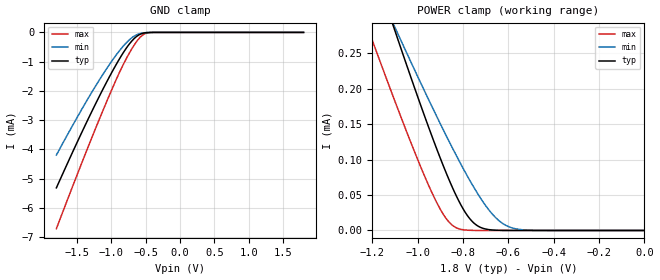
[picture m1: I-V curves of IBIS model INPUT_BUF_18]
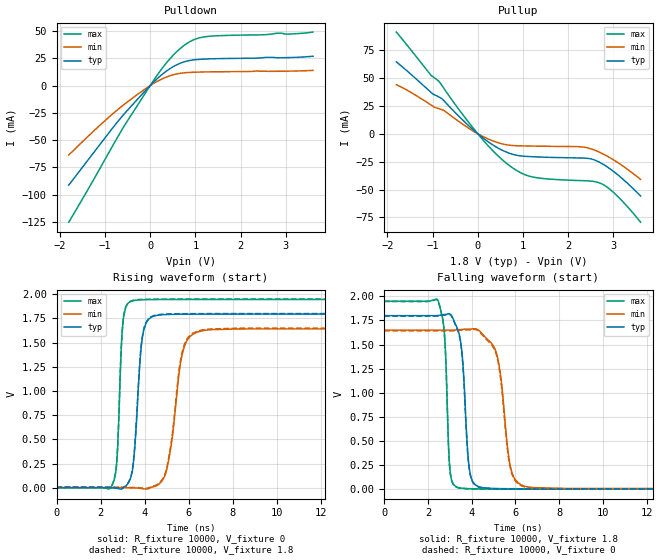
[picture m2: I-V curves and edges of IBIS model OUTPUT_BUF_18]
| TEXAS INSTRUMENTS INCORPORATED
| DLP Products
| IBIS Model of D3664YV2DL
| DLP2000 DMD
| This file contains package information for the following:
|  - LGA 42-pin (PW) package as [Component] DLP2000 DMD
| This device can be powered at the following Vccs:
|  1.8 volt Vcc
| This file provides unique models under the [Model Selector] for each Vcc.
| For operation at a specific Vcc, select the appropriate model after each
| [Model Selector] keyword.
[IBIS Ver]   3.2
[Comment char]  |_char
[File Name]   dlp2000dmd_ibis.ibs
[File Rev]   1.0 | f_die
[Date]   October 20, 2009
[Source]   Data created from TI-SPICE simulations at TI-SLL.
[Notes]   The following is an IBIS list for the P22_NHD.
   Please contact sllibis@ti.com with questions and
   comments concerning SLL IBIS models.
##notes##|
[Disclaimer] Property of Texas Instruments Incorporated.  Unauthorized
   reproduction and/or distribution is strictly prohibited.
   This product is protected under copyright law.
   Created  2009, (C) Copyright  2009, Texas Instruments
   Incorporated, All Rights Reserved
   UNLESS THERE IS A SIGNED, WRITTEN AGREEMENT TO THE
   CONTRARY, TEXAS INSTRUMENTS (TI) IS PROVIDING THE IBIS
   MODELS  AND WITHOUT ANY WARRANTY, EXPRESSED OR
   IMPLIED.  TI assumes no liability for:
   1) the accuracy of the IBIS models provided to your
   company;
   2) the proper functioning of these IBIS Models in your
   design or for any resulting applications; or
   3) infringement of patents, copyrights or intellectual
   property rights resulting from your use of these IBIS
   models.
   TI provides IBIS Models as a service to our customers.
   You and your company shall not distribute, sell or give
   these models to anyone else without prior written
   permission from TI.
   TI reserves the right to make changes to our products or
   to discontinue any semiconductor product or service
   without notice, and advises our customers to obtain the
   latest version of relevant information to verify, before
   placing orders, that the information being relied on is
   current.
   Please be aware that your receipt and use of the IBIS
   information provided shall serve as acceptance of these
   terms and conditions.  If you do not accept these terms,
   you should return or destroy the IBIS models and any
   other accompanying information immediately.
| Component DLP2000 42-pin - LGA
[Component]   DLP2000
[Manufacturer]   Texas Instruments, Inc.
[Package]
|   typ   min   max
R_pkg   6.280e-01   1.680e-01   1.260e+00
L_pkg   5.240e-09   2.810e-09   7.630e-09
C_pkg   2.160e-12   1.040e-12   4.000e-12
[Pin]   signal_name   model_name   R_pin   L_pin   C_pin
1   VCC   POWER
2   D<1>   INPUT_BUF
3   VSS   GND
4   D<2>   INPUT_BUF
5   VSS   GND
6   D<3>   INPUT_BUF
7   D<4>   INPUT_BUF
8   D<5>   INPUT_BUF
9   VSS   GND
10   D<7>   INPUT_BUF
11   VCC   POWER
12   D<6>   INPUT_BUF
13   D<0>   INPUT_BUF
14   VSS   GND
15   DAD_STROBE INPUT_BUF
16   VBIAS   POWER
17   VSS   GND
18   VSS   GND
19   VSS   GND
20   VRESET   POWER
21   VCC   POWER
22   VCC   POWER
23   D<9>   INPUT_BUF
24   VSS   GND
25   D<8>   INPUT_BUF
26   VSS   GND
27   D<11>   INPUT_BUF
28   D<10>   INPUT_BUF
29   VSS   GND
30   DCLK   INPUT_BUF
31   LOADB   INPUT_BUF
32   VCC   POWER
33   SCTRL   INPUT_BUF
34   VSS   GND
35   DAD_BUS   INPUT_BUF
36   VOFFSET   POWER
37   SAC_BUS   INPUT_BUF
38   VSS   GND
39   DAD_OEZ   INPUT_BUF
40   VSS   GND
41   SCAN_TEST  OUTPUT_BUF
42   VCC   POWER
| Model INPUT_BUF
[Model Selector]   INPUT_BUF
INPUT_BUF_18   1.8 volt Vcc
| Model OUTPUT_BUF
[Model Selector]   OUTPUT_BUF
OUTPUT_BUF_18   1.8 volt Vcc
| Models and submodels in the file (2): INPUT_BUF_18 (Input), OUTPUT_BUF_18 (Output)
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[Model]   INPUT_BUF_18
Model_type  Input
Vinl = 0.55
Vinh = 1.25
| variable   typ   min   max
C_comp   0.28pF   0.24pF   0.33pF
[Temperature Range]   40   100   -40
| Ambient temperature   25   85   -40
[Voltage range]   1.8   1.65   1.95
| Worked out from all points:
|   GND clamp passes 1 mA (typ) near -0.90 V on its own axis
[GND Clamp]
| INPUT_BUF_18
|   Voltage   I(typ)   I(min)   I(max)
-1.8V     -5.319mA   -4.198mA   -6.715mA
-1.555V   -4.052mA   -3.147mA   -5.216mA
-1.335V   -2.953mA   -2.248mA   -3.902mA
-1.14V    -2.026mA   -1.501mA   -2.773mA
-970mV    -1.27mA    -905.4uA   -1.833mA
-850mV    -785.1uA   -536.1uA   -1.214mA
-735mV    -390.1uA   -249.6uA   -697.8uA
-640mV    -155uA     -91.95uA   -339.3uA
-555mV    -40.52uA   -24.77uA   -113.2uA
-485mV    -8.678uA   -6.212uA   -26.14uA
-385mV    -582.9nA   -605.8nA   -1.321uA
1.8V      14.91pA    71.9pA     7.535pA
[POWER Clamp]
| INPUT_BUF_18
|   Voltage   I(typ)   I(min)   I(max)
-1.8V     972.9uA    792.1uA    806.9uA
-1.22V    396.3uA    370.8uA    285.3uA
-1.11V    290.7uA    293.1uA    190.3uA
-1.095V   276.5uA    282.7uA    177.6uA
-930mV    126.7uA    170.1uA    48.3uA
-875mV    81.58uA    134.2uA    17uA
-830mV    48.86uA    105.9uA    3.835uA
-785mV    22.91uA    79.02uA    514nA
-740mV    7.387uA    54.23uA    58.41nA
-670mV    665.1nA    22.78uA    1.924nA
-600mV    46.87nA    5.494uA    79.22pA
-16.28fV  14.91pA    56.35pA    10.18pA
[Model]   OUTPUT_BUF_18
Model_type  Output
Vref =   0
Rref =   10000
Cref =   0p
Vmeas =   1.3
| variable   typ   min   max
C_comp   2.96pF   1.27pF   4.57pF
| C_pullup   3.58pF   2.00pF   4.57pF
| C_pulldown   2.33pF   1.27pF   3.11pF
[Temperature Range]   40   100   -40
| Ambient temperature   25   85   -40
[Voltage range]   1.8   1.65   1.95
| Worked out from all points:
|   slope of the pulldown table from 0 to 0.27 V, typ, clamps not added: 25.8 ohm
|   slope of the pullup table from 0 to 0.27 V, typ, clamps not added: 32.4 ohm
|   rising waveform, R_fixture 10000, V_fixture 0: 20-80 % time 305ps typ, 524ps min, 198ps max; typ from 0 V to 1.79 V
|   falling waveform, R_fixture 10000, V_fixture 1.8: 20-80 % time 281ps typ, 469ps min, 184ps max; typ from 1.8 V to 0.004 V
|   rising waveform, R_fixture 10000, V_fixture 1.8: 20-80 % time 304ps typ, 520ps min, 198ps max; typ from 0.004 V to 1.8 V
|   falling waveform, R_fixture 10000, V_fixture 0: 20-80 % time 281ps typ, 471ps min, 184ps max; typ from 1.79 V to 0 V
[Pulldown]
| OUTPUT_BUF_18
|   Voltage   I(typ)   I(min)   I(max)
-1.8V     -91.25mA   -63.67mA   -125.3mA
-840mV    -39.47mA   -26.31mA   -56.03mA
-565mV    -25.58mA   -16.97mA   -36.48mA
-120mV    -5.302mA   -3.372mA   -7.773mA
325mV     12.27mA    7.296mA    19.04mA
530mV     17.85mA    10.17mA    28.75mA
725mV     21.45mA    11.64mA    36.07mA
980mV     23.7mA     12.31mA    42.37mA
1.265V    24.48mA    12.59mA    45.08mA
2.805V    25.53mA    13.16mA    48.04mA
3.145V    25.82mA    13.34mA    47.48mA
3.6V      26.97mA    13.99mA    49.11mA
[Pullup]
| OUTPUT_BUF_18
|   Voltage   I(typ)   I(min)   I(max)
-1.8V     64.38mA    43.84mA    91.09mA
-1.035V   37.09mA    25.85mA    52.39mA
-850mV    32.74mA    22.35mA    46.57mA
50mV      -1.674mA   -1.116mA   -2.446mA
370mV     -10.96mA   -6.967mA   -16.74mA
670mV     -17.03mA   -10.08mA   -27.61mA
955mV     -19.87mA   -10.84mA   -35.05mA
1.22V     -20.6mA    -11.05mA   -38.8mA
2.305V    -21.74mA   -11.79mA   -42.01mA
2.725V    -26.26mA   -17.19mA   -44.6mA
3.09V     -36.62mA   -25.7mA    -56mA
3.6V      -55.75mA   -40.87mA   -79.24mA
[Ramp]
| OUTPUT_BUF_18
| variable   typ   min   max
dV/dt_r   1.09/3.16E-10   0.99/5.33E-10   1.18/2.04E-10
dV/dt_f   1.09/2.93E-10   0.99/4.87E-10   1.18/1.94E-10
R_load = 10000
[Rising Waveform]
| OUTPUT_BUF_18
R_fixture =   10000
C_fixture =   0
L_fixture =   0
V_fixture =   0
V_fixture_min = 0
V_fixture_max = 0
|   Time   V(typ)   V(min)   V(max)
0s        1.19nV     1.938nV    782pV
2.56ns    -2.633mV   20.59uV    43.46mV
2.755ns   -7.516mV   96.76uV    331.5mV
3.025ns   -4.739mV   149.1uV    1.726V
3.42ns    147.6mV    -2.787mV   1.929V
3.88ns    1.523V     -9.578mV   1.942V
4.39ns    1.771V     9.462mV    1.945V
5.77ns    1.793V     1.434V     1.946V
6.405ns   1.794V     1.61V      1.946V
24.99ns   1.795V     1.643V     1.946V
[Falling Waveform]
| OUTPUT_BUF_18
R_fixture =   10000
C_fixture =   0
L_fixture =   0
V_fixture =   1.8
V_fixture_min = 1.65
V_fixture_max = 1.95
|   Time   V(typ)   V(min)   V(max)
0s        1.8V       1.65V      1.95V
2.475ns   1.801V     1.65V      1.95V
2.765ns   1.812V     1.65V      1.58V
3.015ns   1.816V     1.65V      185.9mV
3.375ns   1.651V     1.653V     16.94mV
3.885ns   228.4mV    1.659V     5.233mV
4.355ns   23.29mV    1.642V     3.298mV
5.155ns   6.539mV    1.394V     3.026mV
6.38ns    4.171mV    33.2mV     3.04mV
24.99ns   4.122mV    6.052mV    3.007mV
[Rising Waveform]
| OUTPUT_BUF_18
R_fixture =   10000
C_fixture =   0
L_fixture =   0
V_fixture =   1.8
V_fixture_min = 1.65
V_fixture_max = 1.95
|   Time   V(typ)   V(min)   V(max)
0s        4.12mV     6.048mV    3.007mV
2.56ns    1.473mV    6.068mV    47.34mV
2.75ns    -3.068mV   6.143mV    321.2mV
3.025ns   375.4uV    6.198mV    1.733V
3.42ns    155.8mV    3.229mV    1.933V
3.875ns   1.529V     -3.162mV   1.946V
4.385ns   1.777V     16.57mV    1.949V
5.74ns    1.799V     1.432V     1.95V
6.385ns   1.799V     1.618V     1.95V
24.99ns   1.8V       1.65V      1.95V
[Falling Waveform]
| OUTPUT_BUF_18
R_fixture =   10000
C_fixture =   0
L_fixture =   0
V_fixture =   0
V_fixture_min = 0
V_fixture_max = 0
|   Time   V(typ)   V(min)   V(max)
0s        1.795V     1.643V     1.946V
2.475ns   1.796V     1.643V     1.946V
2.765ns   1.806V     1.643V     1.571V
3.015ns   1.81V      1.643V     179.2mV
3.375ns   1.642V     1.646V     13.74mV
3.88ns    224.4mV    1.652V     2.248mV
4.35ns    19.06mV    1.635V     293.6uV
5.145ns   2.442mV    1.382V     18.56uV
6.37ns    50.17uV    26.6mV     32.69uV
24.99ns   1.322uV    3.772uV    268.6nV
